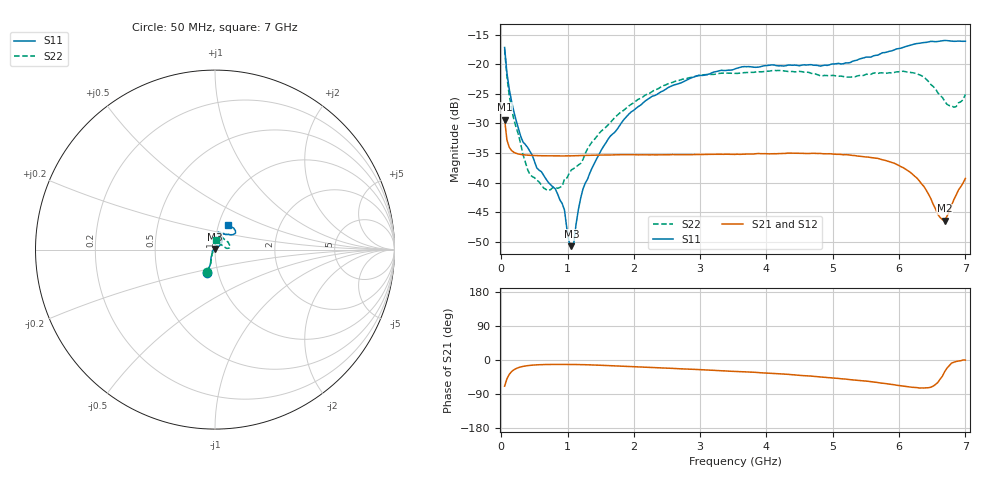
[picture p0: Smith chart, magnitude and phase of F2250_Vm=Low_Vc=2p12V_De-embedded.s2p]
! Integrated Device Technology
! Corporate Headquarters
! 6024 Silver Creek Valley Road
! San Jose, CA 95138  USA
! Phone:  1-408-284-8200
! Toll Free:  1-800-223-1366
! Webpage:  http://www.idt.com/
! Timing and RF Division
! 515 Groton Road, Suite 102
! Westford, MA 01886-6024
! Device:  F2250
! Description: Voltage Variable RF Attenuator
! Frequency:  50.0 -  6000.00 MHz
! Package:  3x3 mm Thin QFN Plastic Package: 16 pin
! Ports:  2 RF, 3 DC
!  Pin  1  = GND
!  Pin  2  = NC
!  Pin  3  = RF1  = Port 1
!  Pin  4  = NC
!  Pin  5  = GND
!  Pin  6  = GND
!  Pin  7  = GND
!  Pin  8  = GND
!  Pin  9  = NC
!  Pin 10  = RF2  = Port 2
!  Pin 11  = NC
!  Pin 12  = GND
!  Pin 13  = GND
!  Pin 14  = VCNTRL
!  Pin 15  = VDD
!  Pin 16  = VMODE
! Vcntrl:  2.120 Volts
! Vmode:  +0.000 Volts
! Vdd:  +3.30  Volts
! Current:  1.180 mA
! Data:  The device was measured on a the F2250 evaluation board which has
!  individual transmission lines to the RF pins.  Data was collected
!  using a calibrated network analyzer.  The evaluation board was
!  de-embedded using a TRL calibration technique.
!  The reference plane is the edge of the package pin.
! Misc:  SN 10
!  Action Tracker AT0258
! Date Measured:  2014-11-26
! Date:  2015-10-15  MJV
! Note:
!  Integrated Device Technology supplies this data as a sample of measured
!  data at the package pin for this product.  Your particular data for this
!  product may vary.
!  Data was taken at 25 degrees C.
!  Integrated Device Technology reserves the right to change this data at anytime.
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# GHz S dB R 50
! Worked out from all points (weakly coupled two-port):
!   201 points, 50 MHz to 7 GHz, reference 50 ohm
!   highest |S21| = -29.35 dB at 50 MHz (marker M1); lowest = -46.5 dB at 6.687 GHz (marker M2)
!   lowest |S11| = -50.8 dB at 1.058 GHz (marker M3), VSWR 1.01, Z = 49.8 + j0.242 ohm
!   |S11| at or under -10 dB: start of sweep to end of sweep
!   |S22| runs from -41.4 to -17.5 dB; largest |S21 - S12| = 5.6e-05
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0.05  -17.18 -108.6  -29.35 -69.1  -29.35 -69.1  -17.52 -109.8
0.08475  -21.44 -107.4  -32.80 -49.7  -32.80 -49.7  -22.10 -107.4
0.189  -28.00 -119.6  -34.89 -25.9  -34.89 -25.9  -29.32 -120.4
0.29325  -32.21 -127.7  -35.26 -18.3  -35.25 -18.3  -33.51 -127.9
0.43225  -34.73 -144.7  -35.41 -14.2  -35.40 -14.2  -38.68 -160.7
0.71025  -39.99 -168.3  -35.49 -11.8  -35.49 -11.8  -41.37 148.1
0.91875  -43.56 158.0  -35.51 -11.6  -35.51 -11.6  -40.62 115.8
0.9535  -44.67 169.8  -35.51 -11.6  -35.50 -11.6  -39.39 115.4
1.023  -50.03 144.1  -35.49 -11.7  -35.49 -11.7  -38.48 96.9
1.05775  -50.76 123.0  -35.49 -11.7  -35.49 -11.7  -37.86 91.9
1.0925  -50.39 90.0  -35.48 -11.8  -35.48 -11.8  -37.64 86.6
1.162  -44.62 56.7  -35.46 -12.0  -35.46 -12.0  -37.04 75.6
1.2315  -41.10 44.1  -35.43 -12.2  -35.43 -12.3  -36.13 67.3
1.6485  -32.11 42.0  -35.35 -14.8  -35.34 -14.8  -29.82 55.3
2.37825  -24.87 47.3  -35.31 -20.6  -35.31 -20.6  -24.07 52.2
3.525  -20.80 72.5  -35.25 -29.9  -35.25 -30.0  -21.57 72.4
4.7065  -20.17 72.4  -35.06 -43.1  -35.06 -43.0  -21.62 71.0
5.85325  -17.82 40.4  -36.47 -63.7  -36.48 -63.7  -21.44 20.5
6.33975  -16.40 41.0  -40.24 -73.7  -40.24 -73.8  -21.95 6.4
6.68725  -15.99 48.8  -46.47 -30.9  -46.44 -30.5  -26.23 26.4
6.861  -16.12 55.1  -42.11 -3.8  -42.07 -3.7  -27.17 58.2
7  -16.12 63.3  -39.31 -0.2  -39.29 -0.2  -25.11 84.9
